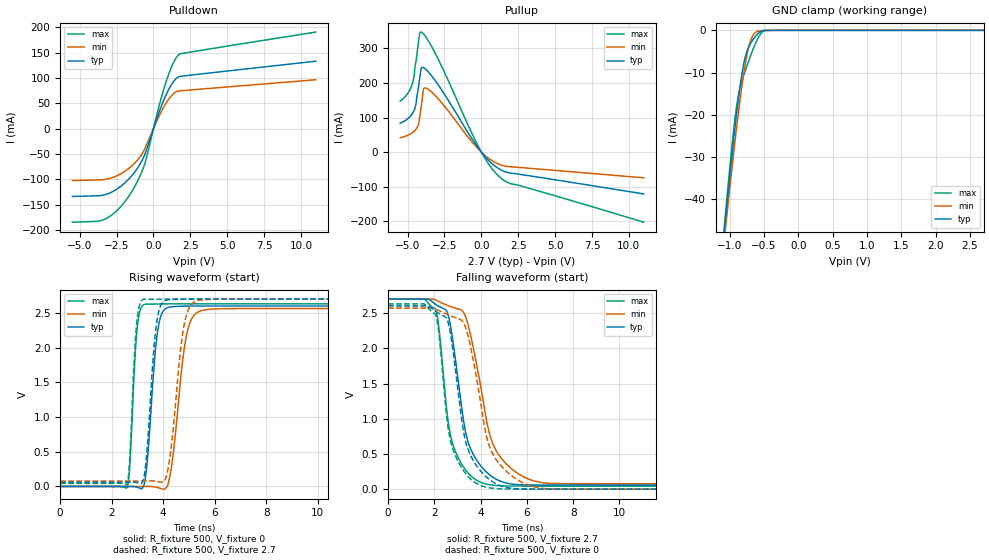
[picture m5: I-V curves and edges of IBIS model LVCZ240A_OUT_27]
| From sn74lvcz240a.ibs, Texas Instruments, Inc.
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[Model]   LVCZ240A_OUT_27
Model_type  3-state
Enable   Active-Low
Vref =   0
Rref =   500
Cref =   30p
Vmeas =   1.35
| variable   typ   min   max
C_comp   4.59pF   NA   NA
| C_pullup   6.27pF   4.53pF   7.32pF
| C_pulldown   5.85pF   5.03pF   7.50pF
| C_tri-state   4.59pF   3.85pF   5.63pF
[Temperature Range]   40   100   -40
| Ambient temperature   25   85   -40
[Voltage range]   2.7   2.7   2.7
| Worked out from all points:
|   slope of the pulldown table from 0 to 0.405 V, typ, clamps not added: 11.8 ohm
|   slope of the pullup table from 0 to 0.405 V, typ, clamps not added: 19.9 ohm
|   GND clamp passes 1 mA (typ) near -0.60 V on its own axis
|   rising waveform, R_fixture 500, V_fixture 0: 20-80 % time 314ps typ, 443ps min, 212ps max; typ from 0 V to 2.6 V
|   falling waveform, R_fixture 500, V_fixture 2.7: 20-80 % time 779ps typ, 1.01ns min, 627ps max; typ from 2.7 V to 0.059 V
|   rising waveform, R_fixture 500, V_fixture 2.7: 20-80 % time 301ps typ, 424ps min, 205ps max; typ from 0.059 V to 2.7 V
|   falling waveform, R_fixture 500, V_fixture 0: 20-80 % time 754ps typ, 958ps min, 618ps max; typ from 2.6 V to 0 V
[GND Clamp]
| LVCZ240A_OUT_27
|   Voltage   I(typ)   I(min)   I(max)
-5.5V     -895mA     -842.7mA   -981.5mA
-1.075V   -46.91mA   -49.02mA   -45.87mA
-1.05V    -42.78mA   -45.14mA   -41.38mA
-950mV    -26.98mA   -30.15mA   -24.71mA
-885mV    -17.71mA   -21.07mA   -16.46mA
-810mV    -9.123mA   -11.75mA   -11.35mA
-745mV    -4.811mA   -5.445mA   -8.233mA
-690mV    -2.92mA    -2.152mA   -5.76mA
-625mV    -1.415mA   -510.5uA   -3.1mA
-550mV    -283.2uA   -115.3uA   -858.6uA
-480mV    -13.06uA   -50.96uA   -17.85uA
2.7V      16.47pA    161.6pA    380.5pA
[Pulldown]
| LVCZ240A_OUT_27
|   Voltage   I(typ)   I(min)   I(max)
-5.5V     -133.6mA   -102.3mA   -184.5mA
-3.81V    -132.3mA   -101.2mA   -182.7mA
-3.235V   -129.8mA   -100mA     -177.6mA
-2.38V    -117.3mA   -91.59mA   -158.8mA
-1.545V   -95.27mA   -75.29mA   -127.6mA
-1.075V   -77.51mA   -61.54mA   -103.1mA
-615mV    -52.9mA    -41.21mA   -71.57mA
335mV     28.73mA    21.91mA    39.57mA
805mV     63.45mA    47.93mA    87.97mA
1.305V    90.79mA    67.52mA    127.2mA
1.735V    102.6mA    74.45mA    146.2mA
11V       133mA      96.4mA     190.5mA
[Pullup]
| LVCZ240A_OUT_27
|   Voltage   I(typ)   I(min)   I(max)
-5.5V     83.27mA    41.43mA    147.5mA
-4.825V   103.3mA    52.26mA    181.9mA
-4.635V   114.4mA    57.55mA    204.5mA
-4.53V    123.9mA    61.43mA    234mA
-4.29V    180.5mA    76.82mA    310.1mA
-4.19V    210.5mA    98.54mA    341.7mA
-4.055V   243.8mA    138.4mA    346.5mA
-3.91V    243.7mA    183.4mA    341.1mA
-3.535V   229mA      179.6mA    317.4mA
-145mV    8.225mA    6.302mA    11.58mA
1.285V    -50.44mA   -36.68mA   -73.69mA
11V       -120.9mA   -74.31mA   -202.6mA
[Ramp]
| LVCZ240A_OUT_27
| variable   typ   min   max
dV/dt_r   1.58/3.26E-10   1.56/4.54E-10   1.59/2.23E-10
dV/dt_f   1.58/7.81E-10   1.57/1.01E-09   1.59/6.31E-10
R_load = 500
[Rising Waveform]
| LVCZ240A_OUT_27
R_fixture =   500
C_fixture =   0
L_fixture =   0
V_fixture =   0
V_fixture_min = 0
V_fixture_max = 0
|   Time   V(typ)   V(min)   V(max)
0s        149.8pV    3.062nV    24.4nV
2.605ns   -163.6uV   -425.7uV   -7.735mV
2.715ns   403.8uV    -406.7uV   368.4mV
2.98ns    -9.497mV   -430.1uV   2.235V
3.275ns   49.47mV    263.7uV    2.623V
3.79ns    2.247V     -15.53mV   2.629V
4.305ns   2.587V     238.3mV    2.631V
4.925ns   2.599V     2.207V     2.631V
5.69ns    2.6V       2.548V     2.631V
50ns      2.601V     2.565V     2.631V
[Falling Waveform]
| LVCZ240A_OUT_27
R_fixture =   500
C_fixture =   0
L_fixture =   0
V_fixture =   2.7
V_fixture_min = 2.7
V_fixture_max = 2.7
|   Time   V(typ)   V(min)   V(max)
0s        2.7V       2.7V       2.7V
2.045ns   2.627V     2.69V      2.557V
2.21ns    2.594V     2.663V     2.253V
2.535ns   2.531V     2.616V     1.122V
2.815ns   2.073V     2.58V      620.1mV
3.41ns    727.6mV    2.39V      247.2mV
4.395ns   201.6mV    773.2mV    62.78mV
5.39ns    70.74mV    274.9mV    44.3mV
7.01ns    59.45mV    81.03mV    43.47mV
50ns      59.15mV    76.97mV    43.24mV
[Rising Waveform]
| LVCZ240A_OUT_27
R_fixture =   500
C_fixture =   0
L_fixture =   0
V_fixture =   2.7
V_fixture_min = 2.7
V_fixture_max = 2.7
|   Time   V(typ)   V(min)   V(max)
0s        59.11mV    76.88mV    43.23mV
2.595ns   60.52mV    76.94mV    38.17mV
2.7ns     61.69mV    77.16mV    392.2mV
2.965ns   56.31mV    77.89mV    2.322V
3.265ns   149.2mV    80.23mV    2.699V
3.74ns    2.337V     73.95mV    2.698V
4.2ns     2.689V     276.2mV    2.7V
4.815ns   2.699V     2.329V     2.7V
5.435ns   2.7V       2.684V     2.7V
50ns      2.7V       2.7V       2.7V
[Falling Waveform]
| LVCZ240A_OUT_27
R_fixture =   500
C_fixture =   0
L_fixture =   0
V_fixture =   0
V_fixture_min = 0
V_fixture_max = 0
|   Time   V(typ)   V(min)   V(max)
0s        2.604V     2.573V     2.632V
2.05ns    2.528V     2.562V     2.48V
2.205ns   2.496V     2.536V     2.185V
2.62ns    2.335V     2.475V     818.5mV
3.24ns    859.2mV    2.375V     273mV
3.61ns    449.5mV    1.951V     130.9mV
4.39ns    134.3mV    598.9mV    19.1mV
5.44ns    8.447mV    165.8mV    916.5uV
6.955ns   323.3uV    3.733mV    242.1uV
50ns      33.06uV    82.44uV    11.91uV
